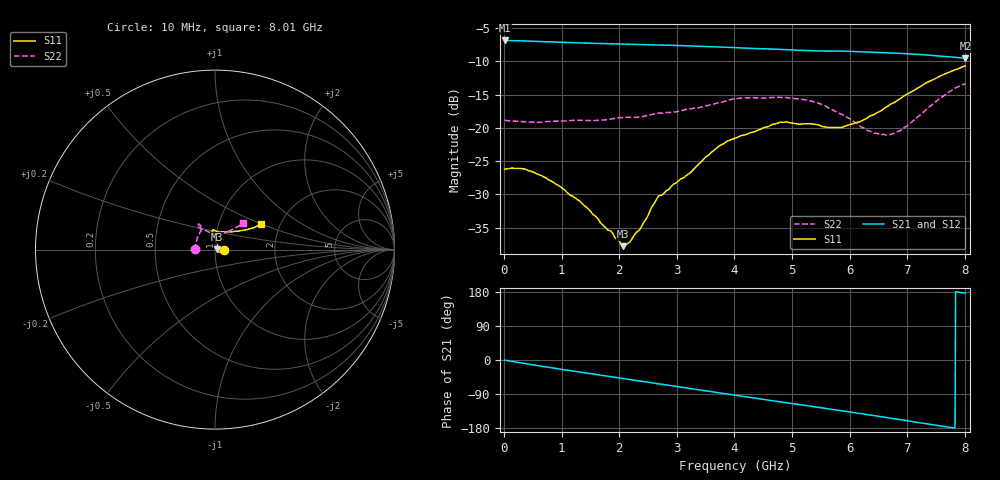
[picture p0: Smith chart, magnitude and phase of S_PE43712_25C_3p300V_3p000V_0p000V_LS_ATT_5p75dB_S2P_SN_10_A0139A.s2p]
! DEVICE ID: PE43712
! File Path: z:\PE43713\PE43713_CHAR_NOM_04292014\AMB\3p300\LS_ATT_5p75dB\PE43713_AMB_3p300V_3p000V_0p000V_LS_ATT_5p75dB_S2P_SN_10_A0139A.s2p
! Serial: 10
! Lot: A0139A
! Temp: 25C
! VDD: 3.300
! VSS: 0.000
! Control_Hi: 3.000
! Control_Lo: 0.000
! Attenuation Step: 5.75dB
! Port 1: RF1
! Port 2: RF2
! ThroughPath:1-2
! IDD: 0.0001472053
! ISS: -1.37e-007
#  Hz  S  RI  R  50
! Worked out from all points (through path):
!   801 points, 10 MHz to 8.01 GHz, reference 50 ohm
!   highest |S21| = -6.87 dB at 10 MHz (marker M1); lowest = -9.5 dB at 8.01 GHz (marker M2)
!   group delay of S21, straight-line fit = 62.9 ps
!   lowest |S11| = -37.8 dB at 2.07 GHz (marker M3), VSWR 1.03, Z = 51.3 + j0.197 ohm
!   |S11| at or under -10 dB: start of sweep to end of sweep
!   |S22| runs from -21.1 to -13.4 dB; largest |S21 - S12| = 0.0014
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1e7  0.0488 -9.45e-05  0.4536 -0.00261  0.4534 -0.00244  -0.1141 0.000662
3.3e8  0.0483 -0.00925  0.4447 -0.067  0.4442 -0.0664  -0.1109 0.0096
6.3e8  0.0416 -0.0141  0.4283 -0.1219  0.4283 -0.1219  -0.1086 0.018
9.6e8  0.0329 -0.0156  0.4028 -0.177  0.4029 -0.177  -0.1087 0.0278
1.35e9  0.0236 -0.0133  0.3659 -0.2341  0.3659 -0.2342  -0.1066 0.0396
2.07e9  0.0127 0.00192  0.28 -0.3217  0.28 -0.3216  -0.0987 0.0677
2.17e9  0.0129 0.0046  0.2664 -0.3318  0.2664 -0.3316  -0.0965 0.0712
2.36e9  0.0125 0.012  0.239 -0.3494  0.239 -0.3492  -0.0903 0.0799
2.68e9  0.0146 0.0268  0.1916 -0.3724  0.1916 -0.3725  -0.0811 0.1003
3.23e9  0.00646 0.0454  0.1038 -0.3991  0.1038 -0.3992  -0.0779 0.1148
3.72e9  0.00128 0.0721  0.0251 -0.4043  0.0249 -0.4043  -0.0798 0.1318
4.01e9  -0.00494 0.0835  -0.0212 -0.4003  -0.0212 -0.4002  -0.088 0.1399
4.79e9  -0.0136 0.1092  -0.1351 -0.3642  -0.1351 -0.3645  -0.0973 0.1387
5.35e9  -0.00149 0.1069  -0.204 -0.3206  -0.2039 -0.3203  -0.0938 0.1274
5.63e9  0.0116 0.0999  -0.2347 -0.2959  -0.2347 -0.296  -0.0783 0.1179
5.87e9  0.0256 0.0975  -0.2619 -0.2711  -0.2614 -0.2712  -0.061 0.11
6.39e9  0.0737 0.0997  -0.3065 -0.2072  -0.3059 -0.207  -0.0158 0.091
6.68e9  0.1075 0.1008  -0.3249 -0.167  -0.3246 -0.167  0.0148 0.0868
6.99e9  0.143 0.1056  -0.3393 -0.1224  -0.3389 -0.1224  0.0459 0.0918
7.35e9  0.1873 0.1148  -0.3453 -0.0687  -0.3449 -0.0686  0.0878 0.1085
7.73e9  0.2289 0.1278  -0.3412 -0.0146  -0.3411 -0.0148  0.1325 0.1317
8.01e9  0.2558 0.1407  -0.3327 0.0201  -0.3321 0.0195  0.1556 0.1467
